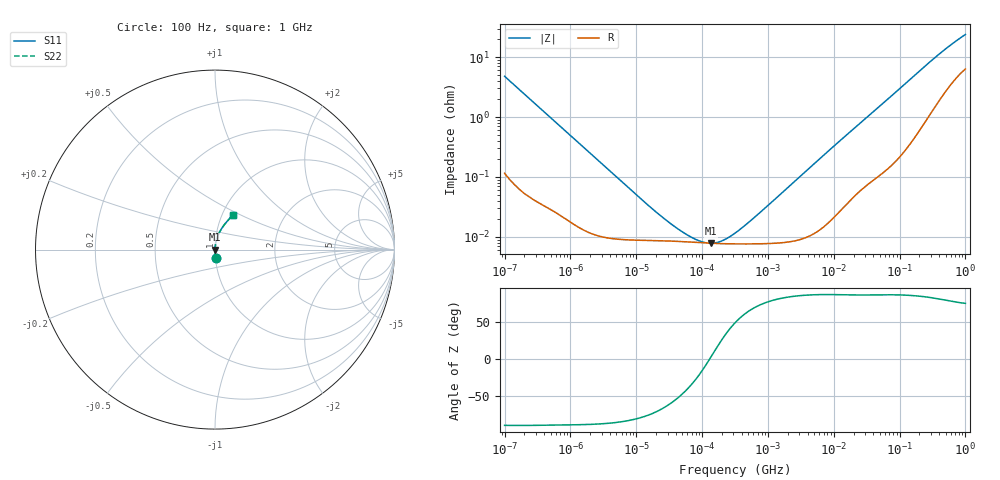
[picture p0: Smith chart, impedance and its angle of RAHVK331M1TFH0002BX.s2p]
! RAHVK331M1TFH0002BX  S-PARAMETER MODEL  (AEC-Q200 qualified)
! Model Generated by ELNA Corporation (http://www.ty-top.com)
! Version 1.0
! ELNA Control No. 240315
! Copyright (c) 2024 ELNA CO.,LTD. All Rights Reserved.
! Products Name : CONDUCTIVE POLYMER HYBRID ALUMINUM ELECTROLYTIC CAPACITORS
! Characteristics :
!  Capacitance  :  330uF  ,  Rated voltage  :  25V
!  Operating Temp. Range  :  -55 to +125 degC  ,  Endurance  :  6000hr at 125 degC
!  Dimension D  :  10mm  ,  Dimension L  :  10mm
! Frequency Range : 100Hz - 1GHz
! External Node Assignments :
!  1  o---| |---o  2
# MHz S RI R 50
!Freq[MHz].  S11 Real  S11 Imag  S21 Real  S21 Imag  S12 Real  S12 Imag  S22 Real  S22 Imag
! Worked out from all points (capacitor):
!   401 points, 100 Hz to 1 GHz, reference 50 ohm
!   read as one part in series: C = 332 uF near 108 Hz
!   lowest |Z| = 7.8 mohm at 135.7 kHz (marker M1)
!   series resonance near 130.1 kHz, so ESL is about 4.5 nH
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0.0001  0.00344 -0.0477  0.9966 0.0477  0.9966 0.0477  0.00344 -0.0477
0.000113  0.00277 -0.0423  0.9972 0.0423  0.9972 0.0423  0.00277 -0.0423
0.000285  0.000691 -0.0169  0.9993 0.0169  0.9993 0.0169  0.000691 -0.0169
0.001488  0.000145 -0.00332  0.9999 0.00332  0.9999 0.00332  0.000145 -0.00332
0.009495  8.82e-05 -0.000521  0.9999 0.000521  0.9999 0.000521  8.82e-05 -0.000521
0.022131  8.61e-05 -0.00022  0.9999 0.00022  0.9999 0.00022  8.61e-05 -0.00022
0.038905  8.43e-05 -0.00012  0.9999 0.00012  0.9999 0.00012  8.43e-05 -0.00012
0.063096  8.18e-05 -6.35e-05  0.9999 6.35e-05  0.9999 6.35e-05  8.18e-05 -6.35e-05
0.074131  8.09e-05 -4.82e-05  0.9999 4.82e-05  0.9999 4.82e-05  8.09e-05 -4.82e-05
0.135675  7.79e-05 3.49e-06  0.9999 -3.49e-06  0.9999 -3.49e-06  7.79e-05 3.49e-06
0.248313  7.64e-05 5.89e-05  0.9999 -5.89e-05  0.9999 -5.89e-05  7.64e-05 5.89e-05
0.280221  7.63e-05 7.2e-05  0.9999 -7.2e-05  0.9999 -7.2e-05  7.63e-05 7.2e-05
0.316228  7.62e-05 8.62e-05  0.9999 -8.62e-05  0.9999 -8.62e-05  7.62e-05 8.62e-05
0.454465  7.61e-05 0.000137  0.9999 -0.000137  0.9999 -0.000137  7.61e-05 0.000137
0.707946  7.64e-05 0.000225  0.9999 -0.000225  0.9999 -0.000225  7.64e-05 0.000225
4.704354  0.000111 0.00154  0.9999 -0.00154  0.9999 -0.00154  0.000111 0.00154
12.8825  0.000296 0.00415  0.9997 -0.00415  0.9997 -0.00415  0.000296 0.00415
69.9842  0.00187 0.0209  0.9981 -0.0209  0.9981 -0.0209  0.00187 0.0209
169.8244  0.00695 0.0492  0.993 -0.0492  0.993 -0.0492  0.00695 0.0492
380.1894  0.0275 0.1014  0.9725 -0.1014  0.9725 -0.1014  0.0275 0.1014
641.9482  0.0605 0.1493  0.9395 -0.1493  0.9395 -0.1493  0.0605 0.1493
1000  0.1018 0.1947  0.8982 -0.1947  0.8982 -0.1947  0.1018 0.1947
